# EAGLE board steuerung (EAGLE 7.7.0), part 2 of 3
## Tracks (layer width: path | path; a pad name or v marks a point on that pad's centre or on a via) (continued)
N$60 (continued)
  Bottom 0.2: 6.9,17.2 6.8,17.2 | 6.8,17.2 6.8,17.1 | 6.8,17.1 6.8,16 7.4,16 7.4,25.4 | 7.4,25.4 7.4,25.6 | 30.1,24.9 30.1,25.6 | 30.1,25.6 7.4,25.6 | 7.4,25.6 7.1,25.6 | 7.1,25.6 7.1,17.4 6.8,17.1 | 6.8,17.2 6.8,25.6 7,25.6 | 7,25.6 7,16.2 6.9,16.1 7.2,16.1 7.3,16.2 7.3,17.1 | 7.3,17.2 7.3,17.1 | 7.3,17.1 7.2,17 | 7.2,17 7.2,16.2 | 7.2,17 7.2,24.6 | 7.2,24.6 7.2,25.2 | 7.2,25.2 7.2,25.4 7.3,25.5 7.1,25.5 7,25.6 | 7,25.6 7.1,25.6 | 30.1,25.6 30,25.5 29.7,25.5 29.7,25.3 | 30.1,25.6 30.3,25.6 30.3,22 | 30.3,22 29.9,22 | 29.9,22 29.7,22 | 29.7,22 29.7,22.3 | 29.7,22.3 29.7,22.7 | 29.7,22.7 29.7,25.1 | 29.7,25.1 29.7,25.3 | 29.7,25.3 29.8,25.2 | 29.8,25.2 29.8,24.7 | 29.8,24.7 29.8,22.4 | 29.8,22.4 29.8,22.1 | 29.8,22.1 29.9,22.1 30,22.2 30,23.2 30.1,23.3 | 30.1,23.3 30.1,22.1 | 30.1,23.3 30.1,24.9 | 30.1,24.9 29.8,25.2 | 29.8,25.4 29.8,25.2 | 29.8,25.2 29.7,25.1 | 29.7,25.1 7.3,25.1 7.2,25.2 | 7.2,25.2 7.4,25.4 | 7.4,25.4 29.9,25.4 | 29.8,22.4 29.7,22.3 | 29.7,22 29.7,21.7 | 29.7,21.7 30.3,21.7 | 30.3,21.7 30.3,22 | 30.3,22 30.2,22.1 30.2,22 30.1,21.9 | 29.8,22.1 29.8,21.9 29.9,21.8 30.1,21.8 | 29.9,22 29.9,21.9 29.7,21.7 | 29.7,21.7 29.7,21.6 | 29.7,21.6 30.3,21.6 30.3,21.7 | 29.3,25.2 29.8,24.7 | 7.2,24.6 7.8,25.2 | 29.9,23 29.9,22.9 29.7,22.7 | 29.7,21.6 29.7,21 29.6,20.9 | 29.6,20.9 25.4,20.9 | 25.3,20.9 25.2,20.9 | 24.8,21.3 24.6,21.5 24.6,22 22.9,22 | 22.9,22 22.9,20.4 24.3,20.4 | IC2.11 7.2,25.2 9.1,25.3 29.96,25.3 IC6.3 30.3,22.55 30.3,21.3 | R5.2 23.62,21.08 23.9,20.8 | 24,20.7 24.3,20.4 | 24.3,20.4 30,20.4 30.1,20.4 30.3,20.6 30.3,21.3 | 30.3,21.3 30.1,21.5 29.9,21.5 29.8,21.4 29.8,20.6 29.9,20.5 | 29.9,20.5 30,20.5 30.1,20.6 30.1,21.3 30,21.4 30,20.7 29.9,20.6
  Bottom 0.2: 29.9,20.6 29.9,20.7 | 29.9,20.7 29.9,20.9 29.6,20.9 | 25.2,20.9 25,20.9 | 25,20.9 23.9,20.9 23.9,20.8 | 23.9,20.8 24,20.7 | 24,20.7 24.2,20.7 | 24.8,20.7 29.9,20.7 | 29.9,20.6 29.9,20.5 | 29.9,20.5 24.4,20.5 24.2,20.7 | 24.2,20.7 24.8,20.7 | 24.8,20.7 25,20.9 | 25,20.9 25,21 24.5,21.5 24.5,20.9 24.6,20.8 24.9,20.8 | 25,20.8 24.9,20.8 | 24.9,20.8 24.4,21.3 24.6,21.3 24.9,21 24.8,21 24.4,21.4 24.4,21.7 24.5,21.8 23.1,21.8 | 23.1,21.8 22.9,22 | 22.9,22 22.9,22.1 | 22.9,22.1 24.7,22.1 | 24.7,22.1 24.8,22 24.8,21.3 | 24.8,21.3 25.2,20.9 | 24.7,22.1 25,22.1 25.1,22 | 25.1,22 25.1,21.2 25.4,20.9 | 25.4,20.9 25.3,20.9 | 25.3,20.9 25,21.2 25,21.9 24.9,22 | 23.1,21.8 23.1,21.9 22.9,22.1 | 22.9,22.1 22.9,22.3 25.1,22.3 25.2,22.2 25.2,21 25.4,20.8 | 25.1,22 25.1,22.2
N$61
  Bottom 0.2: 4.6,18.8 4.3,18.8 4.2,18.9 | 4.2,18.9 4.2,19 | 4.2,19 4.8,19 | 4.8,19 4.8,16 3.5,16 3.5,19 | 3.5,19 3.8,19 | 3.8,19 4.4,19 4.5,18.9 4.5,18.6 | 4.5,18.6 4.5,16.3 4.6,16.2 | 4.6,17 4.6,16.2 | 4.6,16.2 4.7,16.1 3.7,16.1 3.6,16.2 3.6,18.8 3.7,18.9 3.9,18.9 | 4,18.9 4.1,18.9 4.2,18.8 4.2,16.2 4.4,16.2 4.4,18.6 4.3,18.7 4,18.7 | 3.9,18.7 3.8,18.7 3.8,16.3 3.7,16.2 3.9,16.2 4,16.3 4,18.7 | 4,18.7 3.9,18.7 | 3.9,18.7 3.8,18.8 3.7,18.8 3.7,16.6 4.1,16.2 | 4.4,18.7 4.5,18.7 4.8,19 | 4.8,19 4.8,21 3.5,21 3.5,20.7 | 3.5,19 3.5,20.7 | 3.5,20.7 3.7,20.9 4.5,20.9 4.6,20.8 4.6,18.7 4.5,18.6 | 4.5,18.6 4.1,18.6 3.6,19.1 3.6,20.6 3.7,20.7 4.1,20.7 | 4.2,20.7 4.4,20.7 | 4.4,20.7 4.5,20.7 4.7,20.9 4.6,20.9 4.4,20.7 | 4.4,20.7 4.4,19.1 4.2,18.9 | 4.2,19 4.2,20.7 | 4.2,20.7 4.1,20.7 | 4.1,20.7 4,20.8 4,18.9 | 4,18.9 3.9,18.9 | 3.9,18.9 3.8,19 | 3.8,19 3.8,20.6
N$62
  Bottom 0.2: 29.9,24.8 29.8,24.8 29.4,25.2
N$63
  Bottom 0.2: 8.3,17.8 8.3,17.3 8.1,17.1 | 8.1,17.1 8.1,16.2 | 8.1,16.2 8.1,16 8.7,16 8.7,24.5 | 29,23 29,22 | 29,22 28.4,22 | 28.4,23.5 28.4,24 | 28.4,24 28.4,24.5 | 28.4,24.5 28.7,24.5 | 28.7,24.5 29,24.5 29,22.8 28.9,22.7 28.9,24.3 28.8,24.4 28.7,24.4 28.5,24.2 28.5,23.8 28.6,23.7 | 28.6,23.7 28.6,24 | 28.6,24 28.6,24.1 | 28.6,24.1 28.8,24.3 28.8,24.1 | 28.8,24.1 28.8,23.9 | 28.8,23.9 28.8,23.8 | 28.8,23.8 28.7,23.7 28.7,24.5 | 28.4,24.5 8.7,24.5 | 8.7,24.5 8.2,24.5 8.2,16.2 8.3,16.1 8.2,16.1 8.1,16.2 | 8.1,17.1 8.1,24.5 8.4,24.5 8.5,24.4 8.5,24.3 | 8.5,24.3 8.5,16.2 8.6,16.1 8.5,16.1 8.4,16.2 8.4,23.3 8.4,23.4 | 8.4,23.4 8.4,24.4 | IC2.12 8.46,24.07 9.9,24.3 | 9.9,24.3 28.69,24.3 IC6.2 | 8.5,24.3 9.9,24.3 | 28.6,24.1 28,24.1 | 28,24.1 8.6,24.1 8.6,24 28.4,24 | 28.4,24 28.6,24 | 28.6,23.7 28.6,23.2 28.5,23.1 | 28.5,22.9 28.4,22.8 | 28.4,22 28.4,21.7 29,21.7 | 29,21.7 29,22 | 29,22 28.9,22.1 28.7,22.1 28.5,21.9 | 28.5,21.9 28.8,21.9 28.9,21.8 | 28.8,24.1 28.5,24.1 28.4,24 | 28.4,22.8 28.4,22 | 28.4,22.8 28.4,23.5 | 28.4,23.5 28.6,23.7 | 28.6,23.7 28.8,23.9 | 28.8,23.8 28.8,23.2 28.7,23.1 | 29,21.7 29,21.6 28.4,21.6 28.4,21.8 28.5,21.9 | 28.6,23.7 28.4,23.7 28,24.1 | 8.4,23.4 9.2,24.2
N$64
  Bottom 0.2: 27.4,23.3 27.2,23.3 27.1,23.4 | 27.1,23.4 27.7,23.4 27.7,23.3 | 27.7,23.3 27.7,21.7 | 27.7,21.7 26.2,21.7 | 26.2,21.7 26.2,23.3 | 26.2,23.3 26.2,23.4 | 26.2,23.4 26.4,23.4 | 26.4,23.4 26.5,23.4 | 27.7,23.3 27.6,23.2 26.4,23.2 26.3,23.3 26.3,23.1 | 26.3,22 26.3,21.8 27.4,21.8 27.5,21.9 | 27.5,21.9 27.5,22.3 | 27.5,22.3 27.5,22.7 27.4,22.7 27.2,22.9 | 27.2,22.9 27,23.1 26.3,23.1 | 26.3,23.1 26.3,23 | 26.3,23 26.3,22 | 26.3,22 26.4,21.9 27.5,21.9 | 27.5,21.9 27.6,21.8 27.6,22.2 27.5,22.3 | 27.5,22.3 26.4,22.3 26.4,22.2 26.5,22.1 | 26.5,22.1 27.4,22.1 | 26.5,22.1 26.4,22.1 26.4,22.5 | 26.4,22.5 26.4,22.7 26.9,22.7 27,22.8 27,22.5 26.5,22.5 | 26.8,23 26.4,23.4 | 26.2,23.4 9.7,23.4 | 9.7,23.4 9.6,23.4 | 9.6,23.4 9.5,23.3 9.5,16 | 9.5,16 9.4,16 9.4,23.4 9.6,23.4 | 9.7,23.4 9.7,16.2 9.5,16 | 9.5,16 9.9,16 9.9,21.7 | 9.9,23.3 9.9,23.2 | 9.9,23.2 9.9,21.7 | 9.9,21.7 9.6,21.4 9.6,16.3 9.8,16.1 | 27.2,22.9 26.4,22.9 | 26.4,22.9 26.3,23 | 26.3,23 10.3,23 | 10.3,23 9.8,23 9.8,23.1 9.9,23.2 | 9.9,23.2 26.1,23.2 26.3,23 | 26.4,22.9 9.8,22.9 | 26.2,23.3 26.4,23.3 26.5,23.4 | 26.5,23.4 27.1,23.4 | 26.2,21.7 26.2,21.6 27.7,21.6 27.7,21.7 | 25.8,23.1 26.4,22.5 | 9.8,22.4 9.8,22.5 10.3,23
N$65
  Bottom 0.2: 28.7,22.6 28.7,22.3 | 28.7,22.3 28.5,22.1 28.5,22.2 28.6,22.3 28.7,22.3 | 28.7,22.3 28.8,22.2 28.8,22.5
N$66
  Bottom 0.2: 30.2,21.9 30.2,21.8
N$67  (via drill 0.6)
  Bottom 0.2: 12.1,18.6 12.1,18.8 | 12.1,18.8 12.2,18.9 | 12.2,18.9 12.3,19 | 12.4,18.7 12.4,16.9 | 12.4,16.2 12.4,16 11.9,16 11.9,19.1 | 11.9,19.1 12,19.1 | 12,19.1 12.4,19.1 | 12.4,19.1 12.4,19 | 12.4,19 12,18.6 12,16.1 12.3,16.1 12.4,16.2 | 12.4,16.2 12.4,16.9 | 12.4,16.9 12.2,17.1 12.2,16.4 12.1,16.3 12.3,16.3 | 12.1,18.8 12.1,19 12.3,19 | 12.3,19 12.4,19.1 | 12.4,19 12.4,18.7 | 12.4,18.7 12.3,18.6 | 11.9,19.1 11.9,20.4 12.2,20.7 12.9,20.7 | 12.9,20.7 12.9,20 | 12.9,20 12.9,19.9 12.6,19.9 12.4,19.7 | 12.4,19.7 12.4,18.8 12.3,18.7 12.3,19.8 12.5,20 12.6,20 | 12.6,20 12.7,20.1 12.7,20.2 | v12.7,20.3 12.7,20.5 12.8,20.6 12.3,20.6 12.1,20.4 12.1,20 | 12.1,19.3 12.1,20 | 12.1,20 12.2,20.1 | 12.4,20.3 12.6,20.5 12.4,20.5 12.4,20.3 | 12.4,20.3 12.2,20.1 | 12.2,20.1 12.2,19.8 v12.7,20.3 | v12.7,20.3 12.7,20.2 | 12.7,20.2 12.9,20 | 12.9,20 12.6,20 | 12.6,20 12.2,20.4 12.5,20.4 12.6,20.3 12.3,20.3 12.2,20.2 12.3,20.1 | 12.2,19.7 12.2,19.5 | 12.2,19.5 12.2,19.1 | 12.2,18.9 12.2,19.1 | 12.2,19.1 12.1,19.2 | 12,19.4 12,19.1 | 12.2,19.5 12.4,19.7 | 12.4,19.7 13,19.7 13.2,19.9 13.2,20.7 12.9,20.7
N$68
  Bottom 0.2: 11,18.8 11,19.1 | 11,19.1 10.9,19.1 | 10.9,19.1 10.8,19.1 | 10.8,19.1 10.6,19.1 | 10.6,19.1 10.6,16 11.2,16 11.2,19.1 | 11.2,19.1 11,19.1 | 10.9,19.1 10.9,16.4 10.7,16.2 | 10.7,16.2 10.7,17.1 10.9,17.1 11,17 11,16.2 | 10.7,16.2 11,16.2 | 11,16.2 11.1,16.1 | 10.6,19.1 10.6,20.7 | 10.6,20.7 11.2,20.7 11.2,20.4 | 11.2,19.1 11.2,20.4 | 11.2,20.4 11.1,20.5 10.8,20.5 10.8,19.3 11.1,19.3 11.1,20.2 10.7,20.6 | 10.7,20.6 10.7,19.2 10.8,19.1 | 10.8,19.1 10.8,19.9 10.9,20 | 10.9,20 10.9,19.4 | 10.9,20 10.9,20.2 | 10.7,20.6 10.6,20.7 | 10.6,20.7 10.6,22.2 10.7,22.3 12.9,22.3 | 12.9,22.3 12.9,21.3 | 12.9,21.3 12.7,21.3 | 12.7,21.3 11.7,21.3 11.2,20.8 10.8,20.8 10.8,22.1 12.7,22.1 12.8,22.2 12.8,22 | 12.8,22 12.8,21.6 | 12.8,21.6 12.7,21.5 12,21.5 | 12,21.5 11.6,21.5 11.1,21 10.9,21 10.9,21.8 11,21.9 | 11,21.9 12.6,21.9 | 12.6,21.9 12.6,21.7 12.5,21.7 | 12.5,21.7 11.1,21.7 11.1,21.5 | 11.1,21.2 11.2,21.2 11.6,21.6 11.2,21.6 | 11.2,21.6 11.1,21.5 | 11.1,21.5 11.1,21.2 | 11.1,21.2 11,21.1 11,21.9 | 12.6,21.9 12.7,21.9 12.8,22 | 12.8,21.6 12.8,21.4 11.2,21.4 | 11.2,21.4 11.2,21.6 | 11.2,21.6 10.7,22.1 10.7,20.8 11.1,20.4 11.1,20.6 | 12.5,21.7 12.6,21.6 | 11.7,21.6 11.7,21.4 11.2,20.9 11.2,21.4 | 11.1,20.6 11.1,20.7 12,21.6 | 12,21.5 11.1,20.6 | 12.9,22.3 13.2,22.3 13.2,21.3 12.9,21.3 | 12.7,21.3 12.7,21.8 13.1,22.2 13.1,21.5 13,21.4
N$69
  Bottom 0.2: 23.3,14.3 23.2,14.3 23,14.5 22.5,14.5 | 22.5,14.5 22.5,14 25.1,14 | 25.1,14 25.1,14.7 | 25.1,14.7 22.5,14.7 22.5,14.5 | 22.5,14.5 22.7,14.7 24.9,14.7 25,14.6 24.5,14.6 24.1,14.2 | 25.1,14.7 27.4,14.7 27.8,14.4 27.8,12.1 27.4,12.1 27.1,12.4 27.1,13.7 26.8,14 | 26.8,14 25.2,14 | 25.1,14 25.2,14 | 25.2,14 25.4,14.2 26.9,14.2 27.1,14 27.1,12.6 27.4,12.3 27.5,12.3 27.6,12.2 27.6,14.4 27.4,14.6 25.1,14.6 25,14.5 26.8,14.5 27.3,14 | 26.8,14 27.3,14 | 27.3,14 27.3,12.7 | 27.3,12.7 27.5,12.5 27.5,12.8 27.4,12.8 27.3,12.7 | 27.3,12.7 27.3,12.5 27.4,12.4
N$70
  Bottom 0.2: 17.9,12.9 17.6,12.9 17.5,12.8 | 19.5,12.8 20,12.8 | 20,12.8 20,13.3 17.5,13.3 17.5,12.8 | 17.5,12.8 19.5,12.8 | 19.5,12.8 19.9,13.2 19.9,13.1 19.8,13 | 19.5,13 19.8,13 | 19.8,13 20,12.8 | 20,12.8 20.1,12.8 21.3,14 | 21.3,14 21.3,14.4 | 28.1,15.5 28.7,15.2 | 28.7,15.2 28.5,15.2 | 28.5,15.2 28.5,14.9 | 28.5,14.5 28.5,12.4 28.4,12.4 28.4,15.2 28.1,15.5 | IC6.17 28.7,15.2 | 28.7,15.2 28.7,15.5 | 28.1,15.5 27.9,15.5 | 21.3,15.5 21.2,15.5 | 21.2,15.5 21.2,14 20.5,13.3 18.96,13.3 IC4.7 | 28.1,15.5 28.3,15.5 | 28.8,15.5 29,15.5 29,12.1 28.4,12.1 28.4,12.3 28.9,12.3 | 28.9,12.3 28.9,12.2 | 28.9,12.3 28.9,15.4 28.8,15.5 | 28.8,15.5 28.7,15.5 | 28.7,15.5 28.5,15.5 | 28.5,15.5 28.5,15.3 | 28.5,15.3 28.6,15.2 | 28.5,15.3 28.3,15.5 | 28.3,15.5 28.5,15.5 | 28.5,15.5 28.6,15.4 28.6,14.7 | 28.6,14.4 28.6,12.6 28.7,12.5 | 28.7,12.5 28.7,12.6 28.8,12.7 28.8,12.5 28.7,12.4 28.7,12.5 | 21.4,15.5 21.3,15.4 | 21.3,15.4 21.3,15.3 | 21.3,15.2 21.3,15.1 | 21.3,14.4 20.1,13.2 20.1,13 21.1,14 21.1,15.5 21.2,15.5 | 21.3,15.2 21.3,15.3 | 21.3,15.3 21.6,15.5 | 21.3,15.2 21.5,15.2 | 21.5,15.2 21.7,15.5 | 21.7,15.5 22,15.5 | 22,15.5 27.8,15.5 | 27.8,15.5 27.9,15.5 | 27.9,15.5 28.5,14.9 | 28.5,14.9 28.5,14.8 | 28.5,14.8 28.5,14.5 | 28.5,14.5 28.6,14.4 | 28.6,14.4 28.6,14.7 | 28.6,14.7 28.5,14.8 | 27.9,15.4 27.8,15.5 | 21.3,14.4 21.3,15.1 | 21.3,15.1 21.6,15.4 | 21.6,15.4 21.7,15.5 | 21.7,15.5 21.6,15.5 | 21.6,15.5 21.4,15.5 | 21.4,15.5 21.3,15.5 | 21.3,15.5 21.3,15.4 | 21.3,14 21.5,14.2 21.5,15.1 22,15.5 | 21.5,15.2 28.5,15.2 | 21.6,15.4 22,15.4 | 22,15.4 27.9,15.4 | 27.9,15.4 28.5,14.8 | 22,15.4 21.4,14.8
N$83  (via drill 0.6)
  other vias: 11.3,21.8
N$84
  Bottom 0.2: 23.6,14.3 22.6,14.3 22.6,14.1 23.3,14.1 23.4,14.2
N$85
  Bottom 0.2: 70.3,9.1 70.3,11.1 | 70.3,11.7 70.3,12 | 70.3,12 70.3,12.1 69.2,12.1 69.2,12 70.4,10.8 70.4,11.9 70.3,12 | 70.3,12 69.4,12 70.3,11.1 | 70.3,11.1 70.3,11.2 | 70.3,11.6 70.3,11.7 | 70.3,11.7 70.2,11.8 69.7,11.8 70.3,11.2 | 70.3,11.2 70.3,11.5 | 70.3,11.5 70.3,11.6 | 70.3,11.6 70.2,11.7 70.1,11.7 70,11.6 70.2,11.6 70.3,11.5
N$86
  Bottom 0.2: 69.2,14 69.2,12.2
N$87
  Bottom 0.2: 22.6,10.4 22.6,10 22.7,9.9 23.2,9.9 | 23.3,9.9 23.2,9.9 | 23.2,9.9 22.8,10.3 22.8,10.2
N$88
  Bottom 0.2: 28.2,3.7 28.3,3.7 28.9,3.1
N$89
  Bottom 0.2: 34.2,26.6 33.9,26.6 | 33.7,26.6 33.6,26.6 33.6,26 | 33.9,25.5 33.8,25.5 33.7,25.6 33.7,23.3 33.6,23.2 33.8,23.2 33.9,23.3 | IC1.5 46.3,20.84 | 46.3,20.84 46.94,20.84 47,20.9 | 47,20.9 47.1,21 | 47.2,21.1 44.2,21.1 | 44.2,21.1 44.2,21 | 44.2,21 44.2,20.8 | 44.2,20.8 44.2,20.6 47.1,20.6 47.2,20.7 44.6,20.7 44.3,21 44.8,21 | 46.9,21 47.1,21 | 47.1,21 47.2,21.1 | 47.2,21.1 47.2,20.6 44.4,20.6 44.2,20.8 | 44.2,20.8 44.6,20.8 44.8,21 | 44.8,21 46.9,21 | 46.9,21 47,20.9 | 47,20.9 47.1,20.8 44.5,20.8 44.2,21.1 | IC6.6 33.77,23.23 33.5,23.5 | 33.5,23.5 33.5,21.6 34.1,21.6 34.1,23.5 | 34.1,23.5 33.5,23.5 | 33.5,23.5 33.5,25.6 | 33.5,25.6 33.7,25.8 33.9,25.8 | 39.2,25.8 38.5,26.5 34.1,26.5 34.1,23.5 | 39.2,25.8 40.3,24.7 40.3,21 40.4,20.9 42.9,20.9 43.2,20.6 46.06,20.6 46.3,20.84 | 44.2,21.1 44.1,21.1 | 40.8,21.1 40.6,21.3 40.6,24.8 38.7,26.7 33.5,26.7 33.5,26.1 | 33.5,26.1 33.5,25.8 | 33.5,25.6 33.5,25.8 | 33.5,25.8 33.6,25.9 | 33.6,25.9 33.7,26 | 39.2,26 39.3,25.9 39.3,25.8 | 39.3,25.8 40.4,24.7 40.4,24.8 39.4,25.8 39.4,25.7 40.5,24.6 40.5,21.2 40.4,21.1 40.8,21.1 | 40.8,21.1 44.1,21.1 | 44.1,21.1 44.2,21 | 44.2,21 43,21 | 42.9,21 43,21 | 43,21 43.2,20.8 44.2,20.8 | 33.8,23.3 33.9,23.3 | 33.9,23.3 34.1,23.5 | 33.9,23.3 33.9,25.7 | 33.9,25.7 34,25.8 33.9,25.8 | 33.9,25.8 33.8,25.7 | 33.6,25.9 33.6,26 | 33.6,26 33.5,26.1 | 39.2,25.8 39.3,25.8 | 39.3,25.8 39.4,25.9 39.2,25.9 38.5,26.6 38.7,26.6 39.2,26.1 | 33.6,26 33.9,25.7 | 33.9,26 33.9,26.6 | 33.9,26.6 33.7,26.6 | 33.7,26.6 33.7,26 | 33.7,26 33.8,25.9 | 33.9,25.7 33.9,26 | 33.9,26 34.5,26.6
N$90
  Bottom 0.2: 10.8,19 10.8,18.8
N$92
  Bottom 0.2: 51.4,14.3 51.7,14.3 52,14 52,10.9 52.1,10.8 52.2,10.8 52.5,11.1 | 52.5,11.1 52.5,13.9 52.4,14 52.4,11.2 52.3,11.1 52.5,11.1 | 52.5,11.1 52.8,11.4 52.8,13.6 52.7,13.7 52.7,11.5 52.6,11.4 52.9,11.4 53.1,11.6 53.1,13.3 52.9,13.5 52.9,11.7 53,11.6 53.4,12 53.4,12.9 53.3,13 53.3,12.1 53.2,12 53.2,13.1
N$93
  Bottom 0.15: 32.5,22.4 32.4,22.4 32.4,21.8 32.5,21.8 32.5,22.4 | 32.5,22.4 32.6,22.4 | 32.7,22 32.6,22 32.6,22.4 | 32.6,22.4 32.7,22.4 32.7,22.1
N$94
  Bottom 0.2: 59.8,21.6 61.2,23
N$95
  Bottom 0.2: 66,15.4 65.6,15 65.8,15 65.9,15.1 65.5,15.1 65.4,15
N$96
  Bottom 0.2: 32.7,2 35.4,2 35.4,1.8 | 35.4,1.8 35.3,1.7 32.8,1.7 32.7,1.8 32.7,1.9 35.3,1.9 35.4,1.8 | 35.4,1.8 35.4,1.6 | 35.4,1.6 35.4,1.5 32.7,1.5 32.6,1.6 32.6,1.2 35.4,1.2 35.4,1.3 35.3,1.4 32.9,1.4 32.8,1.3 32.8,1.6 32.6,1.8 33.5,1.8 34.2,2.5 | 60.5,12.4 65.5,12.4 65.5,12.6 60.4,12.6 | 67.2,13.8 67.1,13.8 66.1,12.8 | 66,12.7 65.4,12.1 65.4,13.8 | 65.4,13.9 65.4,14.6 65.6,14.6 65.6,12.4 65.8,12.6 65.8,13.3 | 55.7,11.4 60.4,11.4 60.4,11.6 | 60.4,11.6 60.4,12.2 | 60.4,12.2 60.4,13.6 | 60.4,13.6 60.4,14.1 | 60.4,14.1 60.4,14.9 | 60.4,14.9 60.3,14.9 | 60.3,14.9 59.1,14.9 59.1,11.5 | 22.9,8.3 22.9,8.5 23.1,8.7 24.4,8.7 24.7,8.4 24.7,8 24.9,7.8 26.1,7.8 26.5,7.4 | 23.5,7.4 26.5,7.4 | 26.5,7.4 26.7,7.2 | 26.7,7.2 27.3,6.6 31,6.6 31.8,5.8 33.6,5.8 | 34.8,3.81 X1.3 34.7,3.9 34.7,5.3 34.5,5.5 33.9,5.5 | C2.1 65.9,14.7 | 65.9,14.7 63.1,14.7 | 60.55,14.7 IC5.3 | IC5.3 59.8,14.4 60.1,14.7 60.55,14.7 | 60.55,14.7 63.1,14.7 | 63.1,14.7 R2.1 | IC5.3 59.8,12.4 | 59.8,12.4 59.8,11.5 | 59.8,11.5 59.4,11.5 | 59.4,11.5 59.1,11.5 | 59.1,11.5 58.8,11.5 | 58.8,11.5 55.8,11.5 | 55.8,11.5 55.7,11.5 | 55.7,11.5 52.6,8.4 52.7,8.3 52.7,1.3 | R3.2 23.02,7.78 23.7,7.1 26.3,7.1 27.1,6.3 30.8,6.3 31.6,5.5 | 31.6,5.5 31.7,5.5 | 31.7,5.5 33.7,5.5 | 33.6,5.8 33.9,5.5 | 33.9,5.5 33.7,5.5 | 33.7,5.5 33.6,5.6 31.8,5.6 31,6.4 30.9,6.4 | 30.9,6.4 27.4,6.4 | 27.4,6.4 27.2,6.4 26.4,7.2 | 26.4,7.2 26.6,7.2 27.4,6.4 | 26.4,7.2 24.2,7.2 23.7,7.7 23.7,7.5 24,7.2 | 26.7,7.2 26.5,7.2 26.1,7.6 24,7.6 23.9,7.7 23.9,8.6 24.3,8.6 24.4,8.5 24.4,7.8 24.5,7.7 24.9,7.7 24.6,8 24.6,8.4 24.5,8.5 24.5,7.5 24,7.5 23.7,7.2 23.7,8.2 24,8.5 24.2,8.5 24.3,8.4 24.3,8.2 | 24.3,7.7 24.3,8.2
  Bottom 0.2: 24.3,8.2 24.1,8.4 24.1,7.9 24,7.8 24.2,7.8 | 30.9,6.4 30.9,6.3 31.7,5.5 | 31.6,5.5 32.5,4.6 | 32.5,4.6 32.5,2.3 | 32.5,2.3 32.5,2.1 | 32.5,2.1 35.5,2.1 | 35.5,2.1 35.5,3.8 | 35.5,4.2 35.5,4.5 | 35.5,4.5 35.5,4.9 | 35.5,4.9 35.5,5.5 35.4,5.6 32.1,5.6 31.9,5.4 32.6,4.7 32.6,5.4 32.1,5.4 32.4,5.1 | 32.4,5.1 32.4,5.3 | 32.4,5.1 32.4,5 32.5,4.9 32.5,4.6 | 32.5,2.3 32.6,2.2 33.8,2.2 33.8,5.3 33.7,5.4 32.8,5.4 32.7,5.3 32.7,2.3 33.6,2.3 33.7,2.4 32.9,2.4 32.9,5.1 32.8,5.2 33.6,5.2 33.6,2.6 33.7,2.5 33.7,5.2 33.6,5.3 33.2,5.3 33,5.1 33,2.5 33.5,2.5 33.5,5.1 33.3,5.1 | 33.3,5.1 33.2,5.1 33.1,5 33.1,2.7 33.2,2.7 33.3,2.6 33.3,5.1 | 35.5,2.1 35.5,1.3 | 35.5,1.3 35.5,1.1 35.7,1.1 | 35.9,1.1 51.5,1.1 | 51.8,1.1 51.9,1.1 | 51.9,1.1 52.3,1.1 | 52.5,1.1 52.6,1.1 52.7,1.2 | 52.7,1.2 52.7,1.3 | 32.5,2.1 32.5,1 37.8,1 | 38,1 52.8,1 52.9,1.1 52.9,8.5 55.8,11.4 55.8,11.5 | 55.7,11.5 55.6,11.5 52.6,8.5 52.6,1.4 52.3,1.1 | 52.3,1.1 52.5,1.1 | 52.5,1.1 52.7,1.3 | 52.7,1.2 52.7,1.1 | 59.8,11.5 60.2,11.5 60.3,11.6 60.3,12.6 | 60.3,12.6 60.3,14.9 | 60.4,14.9 60.6,14.9 | 60.6,14.9 60.6,14.5 | 60.6,14.5 60.6,13.8 | 60.6,13 60.6,12.8 | 60.6,12.8 60.6,11.4 | 60.6,11.4 59.5,11.4 59.4,11.5 | 59.4,11.5 59.3,11.6 59.3,13.2 59.4,13.3 60.1,13.3 60.2,13.2 | 60.2,12 60.2,11.7 59.5,11.7 59.5,13 59.7,13 | 59.7,13 60,13 60.2,13.2 | 60.2,13.2 60.2,13.1 | 60.2,13.1 60.2,12 | 60.2,12 60,11.8 60,13.2 59.9,13.2 59.7,13 | 59.7,13 59.7,11.9 59.4,11.6 | 59.8,12.4 59.7,12.4 58.8,11.5 | 60.6,14.9 65.2,14.9 | 65.2,14.9 66.3,14.9 | 60.1,11.6 60.4,11.6 | 60.4,11.6 60.6,11.4 | 60.6,11.4 61.7,11.4 62.3,12 65.6,12 67.4,13.8 | 67.4,13.8 67.4,15.5 65.8,15.5 65.2,14.9 | 65.8,13.3 65.8,14.5
  Bottom 0.2: 65.8,14.5 65.8,14.6 65.9,14.7 | 65.9,14.7 65.9,13.5 | 65.9,12.8 65.9,12.9 | 65.9,13.1 65.9,13.5 | 65.9,13.5 66.1,13.7 | 66.1,13.7 66.5,13.7 | 66.5,13.7 66.7,13.7 | 66.7,13.7 66.8,13.8 | 66.7,13.7 65.9,12.9 | 65.9,12.9 65.9,13.1 | 65.9,13.1 66.3,13.5 66.1,13.5 | 66.1,13.5 66.1,12.8 | 66.1,12.8 66,12.7 | 66,12.7 66.1,12.7 | 66.1,12.7 67.2,13.8 | 67.2,13.8 67.1,13.9 67,13.9 66,12.9 66,13.2 66.5,13.7 | 66.5,13.7 66.2,14 66.2,13.8 66.1,13.7 | 60.4,11.6 61.8,11.6 | 61.8,11.6 61.9,11.7 | 61.9,11.7 62,11.8 | 62,11.8 62.2,12 60.6,12 60.5,12.1 60.5,11.8 62,11.8 | 60.4,12.2 65.6,12.2 | 60.3,12.6 60.4,12.6 | 60.4,12.6 60.6,12.8 | 60.6,12.8 65.7,12.8 65.5,13 60.6,13 | 60.6,13 60.3,13 60.2,13.1 | 60.2,13.1 60.3,13.1 60.5,13.3 65.8,13.3 | 65.8,13.3 65.7,13.2 60.8,13.2 60.6,13 | 60.6,13 60.6,13.4 | 60.6,13.4 60.4,13.6 | 60.4,13.6 66,13.6 66.1,13.5 | 66.1,13.5 60.7,13.5 60.6,13.4 | 60.6,13.4 60.6,13.8 | 60.6,13.8 65.4,13.8 | 65.4,13.8 65.4,13.9 | 65.4,13.9 65.5,14 60.5,14 60.4,14.1 | 60.4,14.1 60.5,14.2 65.4,14.2 65.5,14.1 65.5,14.3 60.5,14.3 60.5,14.4 60.6,14.5 | 60.6,14.5 65.8,14.5 | 35.4,1.6 35.6,1.4 | 35.9,1.1 35.7,1.1 | 35.7,1.1 35.5,1.3 | 33.6,5.8 35.4,5.8 35.6,5.6 | 35.6,5.6 35.6,5.3 | 35.6,5.3 35.6,4.6 | 35.6,4.6 35.6,1.4 | 35.6,1.4 35.8,1.2 | 35.8,1.2 35.9,1.1 | 66.1,12.8 66.1,12.7 | 66.1,12.7 65.6,12.2 | 65.6,12.2 65.6,13.3 66.1,13.8 | 61.6,11.5 61.7,11.5 61.8,11.6 | 62,11.8 67.3,11.8 67.3,12.1 | 67.3,12.1 67.3,13.9 67.4,13.8 | 67.4,13.8 67.4,11.8 65.7,11.8 65.6,11.9 67.2,13.5 67.2,13.2 | 67.2,13.2 67.2,12.1 | 67.2,12.1 67.1,12 66.9,12 | 66,12 65.9,12 65.8,11.9 67.1,11.9 67.2,12 67.2,12.1 | 67.1,13.1 66,12 | 66,12 66.9,12 | 66.9,12 67.1,12.2 67.1,13.1 | 67.1,13.1 67.2,13.2
  Bottom 0.2: 67.2,13.2 67,13.2 65.9,12.1 66.8,12.1 67,12.3 67,12.4 | 67,12.4 67,12.8 66.9,12.8 66.3,12.2 66.7,12.2 66.8,12.3 66.8,12.5 66.9,12.6 66.8,12.6 66.5,12.3 66.9,12.3 67,12.4 | 51.9,1.1 51.9,7.9 55.5,11.5 55.5,11.3 52.1,7.9 52.1,1.3 52.2,1.2 52.2,7.9 52.4,8.1 52.4,1.9 | 52.4,1.9 52.4,1.3 52.2,1.3 52.1,1.2 52.1,1.6 52.4,1.9 | 52.4,1.9 52.3,1.9 51.5,1.1 | 51.5,1.1 51.8,1.1 | 51.8,1.1 52,1.3 | 35.6,5.6 37.3,3.9 | 37.3,3.9 37.3,3.8 37.4,3.7 37.4,3.8 | 37.4,3.8 37.3,3.9 | 37.4,3.8 37.6,3.6 37.6,1.4 38,1 | 38,1 37.8,1 | 37.8,1 37.5,1.3 37.5,3.4 37.4,3.5 | 37.2,3.7 37.1,3.8 | 36.9,4 36.7,4.2 | 36.5,4.4 36.3,4.6 | 36.3,4.6 35.6,5.3 | 35.6,5.3 35.7,5.3 37.5,3.5 37.2,3.5 | 37,3.5 36.9,3.5 | 36.7,3.5 35.6,3.5 35.4,3.7 35.7,3.7 | 37.2,3.7 36.5,3.7 | 36.5,3.7 35.7,3.7 | 35.7,3.7 35.4,4 36.9,4 | 36.9,4 37.1,3.8 | 37.1,3.8 36.4,3.8 | 36.3,3.8 35.5,3.8 | 35.5,3.8 35.5,4.2 | 35.5,4.2 36.7,4.2 | 36.7,4.2 36.5,4.4 | 36.5,4.4 35.6,4.4 35.5,4.5 | 35.5,4.5 35.6,4.6 | 35.6,4.6 36.2,4.6 | 36.3,4.6 36.2,4.6 | 36.2,4.6 36.1,4.7 35.7,4.7 35.5,4.9 | 35.5,4.9 35.6,4.9 35.7,5 35.7,4.6 35.8,4.5 35.8,1.2 | 35.8,1.2 36,1.2 36,3.6 36.2,3.6 36.2,1.2 36.4,1.2 36.4,3.7 36.3,3.8 | 36.3,3.8 36.4,3.8 | 36.4,3.8 36.5,3.7 | 36.5,3.7 36.5,1.2 36.7,1.2 36.7,3.5 | 36.7,3.5 36.9,3.5 | 36.9,3.5 36.9,1.2 37.1,1.2 37.1,3.4 37,3.5 | 37,3.5 37.2,3.5 | 37.2,3.5 37.2,1.3 37.3,1.2 37.4,1.2 37.4,3.5 | 37.4,3.5 37.2,3.7 | 61.5,12.7 61.5,12.1 61.9,11.7 | 61.9,11.7 67.4,11.7 67.4,12 67.3,12.1
N$97
  Bottom 0.2: 61.8,21.1 61.3,20.6
N$98
  Bottom 0.2: 4,5.8 4,7.7 | 4,7.7 3.9,7.7 3.9,5.3 6.1,7.6 6.1,7.7 | 6.1,7.7 4.6,7.7 | 4.1,7.7 4.1,6 | 4.1,5.5 4.1,6 | 4.1,6 5.5,7.5 6,7.5 5.9,7.6 4.7,7.6 | 4.3,7.6 4.1,7.6 4,7.7 | 4,7.7 4.1,7.7 | 4.1,7.7 4.6,7.7 | 4.6,7.7 4.7,7.6 | 4.7,7.6 4.3,7.6 | 4.3,7.6 4.2,7.5 | 4.2,6.4 4.2,5.7 | 4.2,5.6 4.2,5.7 | 4.2,5.7 5.9,7.4 4.4,7.4 4.4,7 | 4.4,7 4.4,6.8 | 4.4,6.6 4.4,6.4 | 4.4,6.4 4.4,6 4.3,5.9 4.3,5.7 6.1,7.7 | 6.1,7.7 5.6,7.3 | 5.1,7.3 4.9,7.3 | 4.7,7.3 4.4,7.3 4.2,7.5 | 4.2,7.5 4.2,6.4 | 4.2,6.4 4.5,6.1 4.5,6.2 5.6,7.3 | 5.6,7.3 5.5,7.3 | 5.5,7.3 5.3,7.3 | 5.3,7.3 4.4,6.4 | 4.4,6.4 4.6,6.4 5.5,7.3 | 5.3,7.3 5.1,7.3 | 5.1,7.3 4.4,6.6 | 4.4,6.6 4.4,6.8 | 4.4,6.8 4.9,7.3 | 4.9,7.3 4.7,7.3 | 4.7,7.3 4.4,7
N$99
  Bottom 0.2: 8.2,6.3 8.2,6 6.5,4.3 6.7,4.3 8.1,5.7 | 8.5,14 8.5,11.1 8.2,10.8 | 8.5,14 8.3,14 | 8.3,14 8.1,14 8.1,10.7 | 8.1,10.7 8.3,10.7 | 8.3,10.7 8.6,10.7 | 8.6,10.7 8.6,14 8.5,14 | 8.3,14 8.3,11.1 8.4,11 | 8.4,11 8.4,10.9 | 8.4,10.9 8.6,10.7 | 8.6,5.4 7.4,4.2 | 8.1,10.7 8.1,5.9 | 8.1,5.4 8.1,5.3 7,4.2 7.3,4.2 8.5,5.4 8.5,10.9 8.4,11 | 8.4,10.9 8.4,10.8 8.3,10.7 | 8.3,10.7 8.3,5.7 | 8.3,5.4 8.3,5.7 | 8.3,5.7 8.1,5.9 | 8.1,5.9 8.1,5.7 | 8.1,5.7 8.1,5.4 | 8.1,5.4 6.9,4.2 7.1,4.2 8,5.1 | 8.6,5.4 8.6,5.2 7.5,4.1 | 8.6,10.7 8.6,5.4
N$100
  Bottom 0.2: 29.7,4.8 29.7,2.8 30.2,2.3 30.2,4.9 29.5,5.6 | 29.5,5.6 29.6,5.6 | 29.6,5.6 30.6,5.6 31,5.2 31,1.1 | 31,1.1 28.9,1.1 | 28.9,1.1 28.9,4.9 29.6,5.6 | 29.5,5.6 29.1,5.6 | 29.1,5.6 28.8,5.6 | 28.8,5.6 28.5,5.3 28.5,4.3 | 28.5,4.3 28.5,1.1 | 28.5,1.1 28.8,1.1 | 28.9,1.1 28.8,1.1 | 28.8,1.1 28.7,1.2 28.7,1.6 | 28.7,5.1 28.7,5.3 | 28.7,5.3 30.7,5.3 30.7,1.8 | 30.7,1.8 30.7,1.3 30.6,1.2 30.8,1.2 30.9,1.3 30.9,5.1 30.5,5.5 30.5,5.1 30.4,5 30.5,5 30.6,4.9 29.2,4.9 29.1,5 | 29.1,5 28.7,5.4 28.7,5.3 | 28.7,5.1 28.7,4.8 | 28.7,4.8 28.7,4.6 | 28.7,4.6 28.7,1.6 | 28.7,1.6 29,1.3 30.5,1.3 30.5,1.7 | 30.5,1.8 30.5,2.3 30.3,2.5 29.9,2.5 | 29.9,2.5 29.5,2.5 29.1,2.1 29.1,1.7 | 29.1,1.7 29.1,1.6 29,1.5 30.6,1.5 30.6,1.7 30.7,1.8 | 30.7,1.8 29.2,1.8 29.1,1.7 | 29.1,1.7 30.5,1.7 | 30.5,1.7 30.5,1.8 | 30.5,1.8 30.6,1.9 29.1,1.9 29,2 29.4,2 29.9,2.5 | 28.5,1.1 28.5,1 31,1 31,1.1 | 31,1.1 30.9,1.2 | 29.1,5 29.1,5.6 | 22.6,11.9 22.5,11.9 22.5,12 | 22.5,12 25.1,12 25.1,11.5 22.5,11.5 | 22.5,11.5 22.5,11.8 24.1,11.8 24.3,11.6 23.73,11.6 | 22.7,11.6 22.6,11.7 | 23.4,11.9 22.6,11.9 | 22.6,11.9 22.5,12 | 22.5,12 22.3,12 22.1,11.8 | 22.2,11.8 22.3,11.8 22.4,11.9 22.4,11.6 | 22.4,11.6 22.5,11.5 | X1.2 28.34,3.77 26,6.2 | 25.9,6.2 21.6,6.2 | 21.6,6.2 21.6,10.7 | 22.3,11.5 22.4,11.6 | 22.4,11.6 22.5,11.6 | 22.7,11.6 23.73,11.6 | 23.73,11.6 IC4.3 | 22.5,11.5 22.3,11.5 | 21.6,10.8 22,11.2 | 22,11.2 22.3,11.5 | 22.4,11.6 22.2,11.8 | 22.2,11.8 22.1,11.8 | 22.1,11.8 22,11.7 22,11.4 | 22,11.2 22,11.4 | 22,11.4 22.2,11.6 | 21.6,10.8 21.6,10.7 | 21.6,10.7 21.5,10.7 | 21.6,10.8 21.5,10.7 | 21.5,10.7 21.5,6.2 21.6,6.2 | 22.7,11.6 22.5,11.6 | 22.5,11.6 21.7,10.8 21.7,6.5 21.8,6.4 | 21.7,6.3 21.8,6.4
  Bottom 0.2: 21.8,6.4 25.6,6.4 | 25.6,6.4 29.2,2.8 | 25.6,6.4 26,6.4 26.6,5.8 | 26.8,5.6 27.4,5 | 27.4,5 28.9,3.5 28.9,3.4 28.8,3.3 28.8,3.4 26,6.2 | 26,6.2 25.9,6.2 | 25.9,6.2 25.8,6.3 | 28.8,5.6 26.8,5.6 | 26.8,5.6 26.6,5.8 | 26.6,5.8 26.6,5.7 26.9,5.4 27.5,5.4 | 28.8,5.4 27.5,5.4 | 27.5,5.4 27.3,5.2 28.6,5.2 28.7,5.1 | 28.7,5.1 27.5,5.1 27.4,5 | 27.4,5 27.7,5 | 27.7,5 28.5,5 28.7,4.8 | 28.7,4.8 28.5,4.8 | 28.5,4.8 27.8,4.8 27.7,4.9 27.7,5 | 28.5,4.8 28.7,4.6 | 28.7,4.6 27.9,4.6 27.8,4.5 28.3,4.5 28.5,4.3 | 28.5,4.3 28.4,4.2 28.4,4.3 27.7,5
N$101
  Bottom 0.2: 9.2,4 9.2,4.1 9,4.3 9,4.4 9.5,4.9 9.5,4.8 9.1,4.4 9.3,4.4 9.3,4.5 9.8,5 | IC2.4 9.73,11.83 9.73,13.97 9.7,14 | 9.7,14 9.4,14 9.4,10.6 | 9.4,10.6 9.9,10.6 | 9.9,10.6 9.9,10.9 | 9.9,10.9 9.9,14 | 9.9,14 9.8,13.9 | 9.8,13.9 9.6,13.9 9.7,14 | 9.7,14 9.9,14 | 9.8,13.9 9.7,13.8 9.5,13.8 9.5,10.8 9.6,10.7 9.8,10.7 | 9.8,10.7 9.8,10.9 | 9.8,10.9 9.8,13.5 9.6,13.7 9.6,10.8 | 9.6,10.8 9.4,10.6 | 9.4,10.6 9.4,4.3 9.8,4.3 9.8,5 | 9.8,5 9.8,10.7 | 9.8,10.9 9.9,10.9 | 9.9,10.6 9.9,4.1 | 9.9,4.1 9.8,4.2 9.6,4.2 9.6,10.8 | JP7.4 9.73,2.33 9.8,2.4 9.8,3.4 9.9,3.5 | 9.9,3.5 9.9,3.1 | 9.9,3.1 9.9,2.4 9.8,2.3 9.6,2.3 9.6,2.8 9.9,3.1 | 9.9,3.5 9.9,4.1 | 9.8,5 9.9,5 10.6,4.3 10.4,4.3 10,4.7 10,4.5 10.1,4.4
N$102
  Bottom 0.2: 11.1,6.3 13.1,4.3 12.8,4.3 11.1,6 11.2,6 12.8,4.4
N$103
  Bottom 0.2: 19.1,19.6 19.3,19.6 19.6,19.3
N$104
  Bottom 0.2: 18.6,6.5 19,6.1 20.6,6.1 21.3,5.4 23.7,5.4 23.8,5.3 23.7,5.3 | 18.4,10.7 17.5,10.7 17.5,10.3 | 17.5,10.3 17.5,9.8 | 17.5,9.8 17.7,9.8 | 17.7,9.8 17.8,9.8 | 17.8,9.8 20,9.8 20,10.7 17.7,10.7 17.6,10.6 17.6,10.2 | 18.6,10.1 19.8,10.1 19.8,10.6 19.9,10.5 19.9,10 17.6,10 17.6,10.2 | 18.6,10.1 18,10.1 | 18,10.1 17.7,10.1 | 17.6,10.2 17.5,10.3 | 25.4,5.6 25.4,5.3 24,5.3 23.8,5.5 | 18,10.1 18,9.6 17.8,9.8 | 17.9,9.3 17.9,9.4 18.6,10.1 | 17.5,9.8 17.5,9.3 18.6,8.2 18.6,6.5 | 18.6,10.1 18.6,6.6 18.9,6.3 20.5,6.3 21.1,5.7 | 21.2,5.6 21.2,5.5 21.1,5.6 21.1,5.7 | 21.1,5.7 21.2,5.6 | 21.3,5.5 21.2,5.6 | 21.2,5.6 22,5.6 | 23.5,3.2 23.5,2.1 25.5,2.1 25.5,5.5 25.5,5.6 | 23.5,4.3 23.5,5 23.2,5.3 22.7,5.3 | 22.6,5.3 21.6,5.3 | 21.2,5.3 20.3,6.2 | 18.4,9.7 18.4,6.7 18.6,6.5 | 17.7,9.8 17.7,9.4 | 17.7,9.4 17.7,9.3 18.3,8.7 18.3,9.6 | 17.6,9.6 17.9,9.6 | 18.3,9.6 18.5,9.6 | 18.3,9.6 17.9,9.6 | 17.9,9.6 17.7,9.4 | 17.7,9.4 18.1,9 18.1,9.2 | 18.1,9.2 18.1,9.4 18.2,9.5 18.2,9.3 18.1,9.2 | 23.5,5.3 23.7,5.3 | 23.7,5.3 23.7,5 | 23.7,3.1 23.7,3.2 | 23.7,3.3 23.7,4.3 | 23.7,4.4 23.7,5 | 23.7,5 23.6,5.1 | 23.6,5.1 23.4,5.3 | 23.6,5.1 23.6,4.8 | 23.6,4.8 23.6,4.3 | 23.6,4 23.6,3.8 | 23.6,3.6 23.6,2.8 23.7,2.7 | 23.9,2.5 23.7,2.7 | 23.7,2.7 23.7,2.3 23.6,2.3 | 21.2,5.3 23.1,3.4 23.1,1.9 25.9,1.9 25.9,5.2 25.5,5.6 | 25.4,5.6 22,5.6 | 22,5.6 21.6,5.2 | 21.6,5.1 21.6,5 23.4,3.2 23.4,2.3 23.3,2.2 23.3,3 23.2,3.1 24.7,3.1 25.7,2.1 25.7,5.2 | 25.7,5.3 25.7,5.2 | 25.7,5.2 25.4,4.9 | 21.2,5.3 21.6,5.3 | 21.6,5.3 23.7,3.2 | 23.7,3.2 23.7,3.3 | 23.7,3.3 21.9,5.1 22.1,5.1 23.6,3.6 | 21.6,5.2 21.9,5.2 | 21.9,5.2 22.2,5.2 | 22.4,5.2 22.9,5.2 | 23.2,5.2 24.2,5.2 24.5,4.9 | 23.6,3.6 23.6,3.8 | 23.6,3.8 22.2,5.2
  Bottom 0.2: 22.2,5.2 22.4,5.2 | 22.4,5.2 23.6,4 | 23.6,4 23.6,4.3 | 23.6,4.3 22.6,5.3 | 22.6,5.3 22.7,5.3 | 22.7,5.3 23.7,4.3 | 23.7,4.3 23.7,4.4 | 23.7,4.4 22.9,5.2 | 22.9,5.2 23.2,5.2 | 23.2,5.2 23.6,4.8 | 23.6,4.8 23.4,4.8 23.2,5 22.8,5 | 22.8,5 22.1,5 21.9,5.2 | 21.6,5.2 21.4,5.2 | 21.6,5.2 21.6,5.1 | 21.6,5.1 23.5,3.2 | 23.5,3.2 23.5,4.3 | 23.5,4.3 22.8,5 | 25.4,5.6 25.5,5.6
N$106
  Bottom 0.2: 18.5,6.9 18.5,6.8 19.1,6.2
N$108
  Bottom 0.2: 5.7,17.6 5.7,16 | 5.7,16 5.9,16 | 5.9,16 6.1,16 6.1,23.2 | 6.1,23.2 5.9,23.4 2.8,23.4 | 2.8,23.4 2.7,23.3 2.7,22.1 2.9,21.9 5.3,21.9 5.6,21.6 5.6,16 5.7,16 | 5.9,16 5.9,22.6 | 5.9,22.6 5.9,22.9 | 5.9,22.9 5.9,23.2 2.9,23.2 2.9,23.1 2.8,23 5.8,23 5.9,22.9 | 5.9,22.9 2.9,22.9 2.8,22.8 5.7,22.8 5.9,22.6 | 5.9,22.6 5.8,22.6 | 2.8,22.6 5.8,22.6 | 5.8,22.6 6,22.4 2.9,22.4 2.8,22.3 5.9,22.3 6,22.2 3.1,22.2 2.8,22.5 2.8,22.1 2.9,22 5.6,22 5.7,21.9 3.1,21.9 2.9,22.1 5.7,22.1 5.8,22 5.8,21.6 | 5.8,18.6 5.8,21.6 | 5.8,21.6 5.6,21.8 | 6.1,23.2 6.1,23.5 | 6.1,23.6 6.1,23.5 | 6.1,23.5 6,23.4 6,23.5 6.1,23.6 | 6.1,23.6 2.6,23.6 2.6,21.9 2.7,21.8 5.3,21.8 5.7,21.4 | 2.8,23.4 2.7,23.5
N$109
  Bottom 0.2: 20,3.1 20,3.3 | 20,3.3 20.8,3.3 | 20,3.3 19.4,3.3 19.9,3.8
N$110
  Bottom 0.2: 17.7,6.3 17.8,6.3 18.7,5.4
N$111  (via drill 0.6)
  Top 0.2: v4.2,22.8 42.1,22.8 v42.1,9.9
  Bottom 0.05: v4.2,22.8 5.8,22.8 IC2.10
  Bottom 0.2: 36.4,13.7 36.4,14.9 36.1,14.9 36.1,13.7 | 36.1,13.7 36.2,13.6 36.2,13.7 | 36.2,13.7 36.2,14.7 36.3,14.8 36.3,13.5 | 36.2,10.8 36.2,12 | 36.2,12 36.2,12.7 | 36.2,12.7 36.3,12.8 36.3,12.6 | 36.4,10.7 36.7,10 | 36.8,10 37.8,9.6 | 37.8,9.6 43.1,9.6 43.1,9.8 43,9.9 37.4,10.2 36.8,10.1 | 36.8,10.1 42.9,9.7 43,9.8 43,9.5 | 36.6,13.6 36.6,15 36,15 36,13.6 | IC6.11 36.6,12.9 36.6,12.5 | 36.6,10.8 36.6,10 | 36.6,10 37.3,10.1 | 37.3,10.1 v42.1,9.9 | 36.6,10.8 37.1,10.3 43,10.3 43.2,10.1 43.2,9.5 43,9.5 | 36.6,10.8 36.6,12.5 | 36.6,12.5 36.4,12.7 36.4,10.7 | 36.4,10.7 36.7,10.4 | 36.7,10.4 36.8,10 | 36.8,10 36.9,10.1 | 36.9,10.1 36.5,10.5 | 36.5,10.5 36.4,10.7 | 36.4,10.7 36.3,12.6 | 36.3,12.6 36.2,12.7 | 43,9.5 37.7,9.5 | 37.7,9.5 36.8,10 | 36.8,10 36.5,10.5 | 36.5,10.5 36.7,10.4 | 36.7,10.4 36.6,10 | 36.6,10 36.7,10 | 36.7,10 36.8,10 | 36.8,10 43.1,10 43,10.1 37.3,10.1 | 37.3,10.1 37.1,10.1 | 37.1,10.1 36.9,10.1 | 36.9,10.1 36.8,10.1 | 36.8,10.1 36.7,10.1 36.7,10.4 | 36.7,10.4 36.8,10.4 | 36.8,10.4 37.1,10.1 | 36.8,10.4 36.7,10.5 36.7,10.4 | 36.7,10.4 36.9,10.2 | 36,13.6 36,12.9 | 36,12.9 36.2,12.7 | 36.2,13.7 36.1,13.7 | 36.1,13.7 36,13.6 | 36,12.9 36,12.2 36.2,12 | 36.2,10.8 36.5,10.5 | 36.9,10.1 37.7,9.5 | 37.7,9.5 37.8,9.6 | 36.2,10.8 36.2,10.4 37.1,9.5 41.3,9.5 41.5,9.7 | 41.5,9.7 37.1,9.7 36.3,10.5 36.4,10.5 37,9.9 41.3,9.9 41.5,9.7
N$112
  Bottom 0.2: 67.2,10.4 67.2,9.9 | 67.2,9.4 67.2,9.1 64.6,9.1 64.2,8.7 | 64.2,8.7 61.3,8.7 59.3,6.7 55.6,6.7 55.6,8.8 | 55.8,9 57.1,10.3 | 57.1,10.3 57.2,10.4 | 57.2,10.4 67.2,10.4 | 66,10.3 67.1,10.3 67.2,10.4 | 67.2,10.4 68.3,10.4 68.6,10.1 68.6,9.1 67.5,9.1 67,8.6 60.7,8.6 | 60.2,8.9 59.9,8.9 59.3,8.3 59.3,8 59.1,7.8 59.4,7.8 60.4,8.8 | 61.4,8.9 61.3,8.9 59.3,6.9 59.3,7.1 | 55.7,8.7 56,9 | 56,9 56.2,9.2 | 56.2,9.2 56.6,9.6 | 56.6,9.6 56.8,9.8 | 56.9,9.9 57.3,10.3 65.9,10.3 66.1,10.1 65.8,10.1 | 57.2,10.1 65.8,10.1 | 65.8,10.1 66,9.9 56.9,9.9 | 56.9,9.9 56.8,9.8 | 56.8,9.8 66,9.8 66,9.6 56.6,9.6 | 56.6,9.6 56.6,9.5 56.5,9.4 66,9.4 65.9,9.3 56.2,9.3 56.2,9.2 | 56.2,9.2 64.6,9.2 64.2,8.8 61,8.8 | 60.4,8.8 56,8.8 56.2,9 60.9,9 | 61.1,9 64.3,9 | 59.3,7.1 59.3,7.2 60.7,8.6 | 60.7,8.6 61.1,9 | 61.1,9 60.9,9 | 60.9,9 59.4,7.5 59.4,7.7 60.6,8.9 60.3,8.9 59.2,7.8 59.2,8 60.1,8.9 59.8,8.9 59.1,8.2 | 60.4,8.8 61,8.8 | 61,8.8 61.1,8.9 | 61,8.8 59.3,7.1 | 64.2,8.7 67,8.7 67.5,9.2 67.5,10.1 67.4,10.2 | 67.4,10.2 68.3,10.2 | 67.4,10.2 65.9,10.2 64.5,8.8 66.8,8.8 67.4,9.4 67.4,9.9 67.3,10 66.1,10 66.1,9.5 65.3,9.5 64.7,8.9 67.1,8.9 67.4,9.2 67.4,10.1 66.5,10.1 66.3,9.9 66.3,9.5 | 66.3,9.5 66,9.2 66.3,9.2 | 66.3,9.2 67,9.2 67.2,9.4 | 67.2,9.4 67.2,9.8 | 67.2,9.8 67.2,9.9 | 67.2,9.9 66.5,9.9 66.4,9.8 66.4,9.3 66.3,9.2 | 66.3,9.2 66.3,9.3 66.5,9.5 67.1,9.5 67.1,9.4 66.3,9.4 66.3,9.5 | 66.3,9.5 66.6,9.8 67.2,9.8 | 56,9 55.8,9 | 55.8,9 55.6,8.8 | 55.6,8.8 55.5,8.7 54.3,8.7 | 54.3,8.7 54.1,8.5 | 54.1,8.5 53.8,8.2 53.8,6.7 56.3,6.7 56.4,6.8 54,6.8 53.9,6.9 53.9,7.7 | 53.9,7.7 53.9,8 54.3,8.4 | 54.3,8.4 54.5,8.6 | 54.6,8.6 55.1,8.6 | 55.1,8.6 56,8.6 | 54.5,8.6 54.4,8.6
  Bottom 0.2: 54.4,8.6 54,8.2 54,8 | 54,8 54,7.9 | 54,7.6 54,7.4 | 54,7.2 54,7 55.8,7 55.9,7.1 55.9,7.2 54,7.2 | 54,7.2 54,7.4 | 54,7.4 56.1,7.4 56.1,7.6 55.8,7.6 | 54,7.6 54,7.9 | 54,7.9 56.4,7.9 56.6,7.7 55.9,7.7 55.8,7.6 | 55.8,7.6 54,7.6 | 54,7.6 53.9,7.7 | 53.9,7.7 56.3,7.7 56.4,7.6 56.2,7.6 55.7,8.1 54.3,8.1 | 54.3,8.1 54.1,8.1 54,8 | 54,8 55.6,8 55.8,8.2 | 54.2,8.2 55.8,8.2 | 55.8,8.2 56,8.4 54.8,8.4 | 54.6,8.4 54.3,8.4 | 54.3,8.3 54.3,8.7 | 54.3,8.1 54.3,8.3 | 54.3,8.3 54.1,8.5 | 54.3,8.7 56,10.4 56.3,10.4 | 57.2,10.4 56.3,10.4 | 56.3,10.4 56.2,10.3 56.1,10.3 54.4,8.6 | 54.5,8.6 54.6,8.6 | 54.6,8.6 56.3,10.3 56.5,10.3 | 57.1,10.3 56.8,10.3 | 56.7,10.3 56.5,10.3 | 56.5,10.3 54.6,8.4 | 54.6,8.4 54.8,8.4 | 54.8,8.4 56.7,10.3 | 56.7,10.3 56.8,10.3 | 56.8,10.3 56.9,10.2 56.7,10.2 55.1,8.6
N$117
  Bottom 0.2: 21.3,18.3 21.3,18.2 21.7,17.8
N$118
  Bottom 0.2: 39.2,5.4 39.2,5.6 37.4,5.6 | 37.4,5.6 37.3,5.7 | 37.4,5.6 37.5,5.5 38.9,5.5 39,5.4 38,5.4 37.9,5.3 38.9,5.3
N$119
  Bottom 0.2: 22.7,0.3 22.6,0.3 20.5,0.4
N$120
  Bottom 0.2: 31,26.4 30.4,26.4 | 30.4,26.4 6.5,26.4 | 6.5,26.4 6,26.4 | 6,26.4 5.9,26.4 | 5.9,26.4 5.7,26.4 5.7,26.5 30.9,26.5 | 5.6,26.7 31.23,26.7 | 31.23,26.7 IC6.4 | 6.1,26.5 6.1,26.2 | 6.4,26.2 30.7,26.2 | 30.7,26.2 31,26.2 31,25.8 | 31,25.8 31,22.2 | 31,22.2 31.5,22.2 | 31.5,22.2 31.5,26.7 31.4,26.7 | 31.4,26.7 31.3,26.6 31.3,26.7 | 31.3,26.7 31.23,26.7 | 31.3,26.7 31.4,26.7 | 31.4,26.7 31.4,26.6 31.3,26.5 31.3,22.4 31.5,22.2 | 31.5,22.2 31.5,22.1 | 31.5,22.1 31.5,22 | 31.5,22 31.4,22 | 31.4,22 30.9,22 | 30.9,22 30.9,26.5 | 30.9,26.5 30.9,26.6 31,26.6 31.1,26.5 31.1,25.8 | 31.1,25.8 31.1,22.4 31.2,22.3 | 6,26.4 5.9,26.3 5.9,25.8 6.5,26.4 | 5.9,26.6 5.7,26.6 5.6,26.7 | 5.6,26.7 5.5,26.7 | 30.9,22 30.9,21.7 | 30.9,21.7 31.5,21.7 | 31.5,21.7 31.5,22 | 31.5,22.1 31.3,22.1 31.1,21.9 | 31,22.2 31,21.9 31.1,21.8 31.4,21.8 | 31.4,22 31.4,21.8 | 31.4,21.8 31.5,21.7 | 31.5,21.7 31.5,21.6 30.9,21.6 30.9,21.7 | 31.1,25.8 30.7,26.2 | 30.4,26.4 31,25.8 | JP1.1 5.5,25.67 5.5,26.7 | 5.5,26.7 2.9,26.7 2.6,26.4 2.6,24.7 6.1,24.7 6.1,25.9 6.4,26.2 | 6.4,26.2 6.1,26.2 | 6.1,26.2 6,26.1 6,24.9 2.7,24.9 2.7,26.3 2.9,26.5 5.8,26.5 5.9,26.4 | 5.9,26.4 5.9,25.1 2.8,25.1 2.8,25.4 | 2.8,26.1 2.8,26.2 3,26.4 5.6,26.4 5.8,26.2 5.8,25.3 5.7,25.2 3,25.2 2.9,25.3 | 2.8,26 2.8,26.1 | 2.8,26.1 2.9,26.2 5.5,26.2 5.6,26.3 5.6,26 5.7,25.9 5.7,25.3 2.9,25.3 | 2.9,25.3 2.8,25.4 | 2.8,25.4 2.8,25.5 | 2.8,25.9 2.8,26 | 2.8,26 2.9,26.1 5.4,26.1 5.5,26 | 5.6,25.8 5.6,25.6 5.5,25.5 2.8,25.5 | 2.8,25.5 2.8,25.9 | 2.8,25.9 2.9,26 5.5,26 | 5.5,26 5.6,25.9 5.6,25.8 | 5.6,25.8 2.9,25.8 2.9,25.6 4.9,25.6 5,25.7 5.3,25.7 5.6,25.4
N$121
  Bottom 0.2: 2.7,21 2.9,21 2.9,14.6 2.4,15.1 2.4,21 2.7,21 | 2.7,21 2.8,20.9 2.8,14.8 | 2.8,14.8 2.9,14.7 | 2.8,14.8 2.5,15.1 2.5,20.8 2.6,20.9 2.6,15.2 2.7,15.1
N$123
  Bottom 0.2: 13.8,14.7 13.8,15.4 3.5,15.4 3.5,14.7 | 13.8,14.7 3.5,14.7 | 3.5,14.7 3.5,14.6 13.8,14.6 | 13.8,14.6 13.7,15 13.8,15.2 3.7,15.3 3.6,15.2 3.6,15.1 13.8,15.1 13.6,14.9 3.7,14.9 3.6,14.8 3.6,14.9 3.7,15 | 13.8,14.7 13.8,14.6
N$124  (via drill 0.6)
  Top 0.2: v44.3,11.4 2.1,11.4 v2.1,6.8
  Bottom 0.05: v2.1,6.8 JP7.1
  Bottom 0.2: 43.7,10.9 43.7,10.8 | 43.7,10.8 43.9,10.6 45.2,10.6 45.2,10.7 | IC6.10 37.9,13.31 | 37.9,13.31 37.9,11.9 | 37.9,11.9 37.9,11.4 v44.3,11.4 | 37.9,14.3 37.9,14.6 37.7,14.8 37.3,14.8 37.3,11.4 37.4,11.3 | 37.6,11.1 43.4,11.1 | 43.6,11.1 44.9,11.1 44.9,11.8 | 44.9,11.8 42.1,11.8 42,11.7 38.1,11.7 37.9,11.9 | 37.9,13.31 37.9,14.3 | 37.9,14.3 37.7,14.5 | 37.7,14.5 37.5,14.7 37.5,11.4 37.7,11.2 44.7,11.2 | 44.7,11.2 44.7,11.5 | 44.7,11.5 37.8,11.5 37.7,11.4 44.5,11.4 44.7,11.2 | 44.7,11.5 44.7,11.6 37.7,11.6 | 37.7,11.6 37.7,14.5 | 37.7,14.7 37.7,14.5 | 37.7,11.6 37.6,11.5 | 44.9,11.8 45.2,11.8 45.2,10.7 | 45.2,10.7 43.8,10.7 43.4,11.1 | 43.4,11.1 43.6,11.1 | 43.6,11.1 43.8,10.9 45.1,10.9 45.1,11.2 | 45.1,11.6 45.1,11.2 | 45.1,11.2 45,11.1 45,11.7 | 37.4,11.6 37.4,11.3 | 37.4,11.3 37.6,11.1 | 37.6,11.1 37.7,11 43.5,11 43.7,10.8
N$125
  Bottom 0.2: 15.6,8.4 16.6,7.4 16.3,7.4 | 14.5,14 14.5,8.3 16.4,6.4 | 16.4,6.4 16.9,6.4 16.9,6.5 | 16.9,7.3 16.9,7.7 | 16.9,7.7 16.7,7.9 | 16.7,7.9 16.1,8.5 16.1,13.9 | 16.1,13.9 14.6,13.9 14.5,14 | 14.5,14 16.1,14 | 16.1,14 15.9,13.8 14.6,13.8 14.6,8.4 16.5,6.5 16.6,6.5 | 16.6,6.5 16.7,6.6 16.7,6.8 | 16.7,7 16.7,7.7 16.1,8.3 16.1,7.3 16.6,6.8 | 16.6,6.8 16.9,6.5 | 16.9,6.5 16.9,7.3 | 16.9,7.3 16.2,8 16.2,7.7 16.6,7.3 16.3,7.3 16.2,7.4 | 16.2,7.4 16.3,7.4 | 16.3,7.4 16.7,7 | 16.7,7 16.7,6.8 | 16.7,6.8 16.6,6.7 14.8,8.5 14.9,8.5 | 15.7,8.5 15.9,8.5 15.9,8.4 | 15.9,8.2 15.9,7.8 15.7,7.8 | 15.7,7.8 15.1,8.4 | 15.1,8.4 15.2,8.4 15.3,8.3 | 16.2,7.4 16.2,7.5 15.4,8.3 15.8,8.3 15.9,8.4 | 15.9,8.4 15.9,8.2 | 15.9,8.2 15.8,8.1 15.7,8.2 15.8,8.2 16,8.4 16,13.6 15.9,13.7 | 15.9,13.7 14.8,13.7 14.8,8.7 | 14.8,8.7 14.8,8.6 14.9,8.5 | 14.9,8.5 15.7,8.5 | 15.7,8.5 15.8,8.6 15.8,8.7 | 15.8,8.7 15.8,13.6 15.5,13.6 | 15.4,13.6 15.3,13.6 | 15.2,13.6 15,13.6 15,8.8 15.4,8.8 15.7,8.5 | 15.7,8.5 15.7,8.6 | 15.7,8.6 15.8,8.7 | 15.8,8.7 15.5,8.7 | 14.8,8.7 14.9,8.7 | 14.9,8.7 15.1,8.7 | 15.1,8.7 15.5,8.7 | 15.5,8.7 15.6,8.8 15.6,9.1 | 15.6,9.1 15.6,13.5 15.5,13.6 | 15.5,13.6 15.4,13.6 | 15.4,13.6 15.3,13.5 15.3,8.9 15.1,8.7 | 15.1,8.7 15.1,9.4 15.2,9.5 15.2,13.6 | 15.2,13.6 15.3,13.6 | 15.3,13.6 15.5,13.4 15.5,8.8 15.7,8.6 | 14.9,8.7 14.9,8.3 | 14.9,8.3 16.5,6.7 | 16.6,6.8 16.6,6.6 16.4,6.4 | 16.4,6.4 17.4,5.4 | 17.4,5.4 17.7,5.1 | 17.7,5.1 17.8,5.1 17.8,5.4 | 17.8,5.4 17,6.2 | 17,6.2 16.7,6.5 | 16.6,6.5 16.6,6.4 17.6,5.4 | 17.6,5.4 17.7,5.3 | 17.6,5.4 17.5,5.4 17.4,5.5 17.4,5.4 | 17.7,5.1 18,4.8 18,5.2 17.8,5.4 | 16.2,7.4 15.3,8.3 | 15.3,8.3 14.9,8.3 | 14.9,8.3 14.8,8.4 15.1,8.4 | 15.7,7.8 16.6,6.9 16.6,7.8 16.7,7.9
  Bottom 0.2: 16.9,7.7 17,7.6 17,6.2 | 15.6,9.1 17,7.7 | 16.1,14 16.1,13.9 | 16.1,13.9 15.9,13.7
N$126
  Bottom 0.15: 33.6,22.4 33.6,21.7 33.7,21.7 | 33.8,21.7 34,21.7 34,22.2 | 33.8,22.3 33.7,22.3 33.7,21.7 | 33.7,21.7 33.8,21.7 | 33.8,21.7 33.8,22.3 | 33.8,22.3 34,22.3 34,22.2 | 34,22.2 33.9,22.2 33.9,21.8
N$127
  Bottom 0.2: 1.5,9.6 1.5,8.6 | 1.5,8.6 1.5,8.5 2,8.5 2.1,8.6 2.1,8.7 | 2.1,9.5 2.1,9.6 2,9.6 | 1.4,9.6 2,9.6 | 2,9.6 2.1,9.5 | 2.1,9.5 2.1,8.7 | 2.1,8.7 2,8.6 1.9,8.6 1.7,8.8 | 1.6,8.9 1.6,8.7 1.8,8.7 2,8.9 2,9.2 | 2,9.2 2,9.4 1.9,9.5 1.7,9.5 1.6,9.4 1.6,8.9 | 1.6,8.9 1.7,8.8 | 1.7,8.8 1.7,9.3 1.8,9.4 1.8,9 | 1.8,8.9 1.8,9 | 1.8,9 2,9.2 | 2.3,9.8 2.3,8.4 1.3,8.4 | 1.3,8.4 1.3,9.8 2.2,9.8 | 1.5,8.6 1.3,8.4 | 1.3,8.4 0.7,8.4 0.7,9.8 1,9.8 | 1.2,9.8 1,9.8 | 1,9.8 0.9,9.7 | 0.9,9.7 0.9,8.5 1.1,8.5 1.1,9.6 1.2,9.7 0.9,9.7
N$129
  Bottom 0.2: 44.9,22 43.2,22 43.1,22.1 | 43.1,22.1 43,22.1 | 43.1,22.1 44.7,22.1 44.8,22.2
N$130
  Bottom 0.2: 19,5.2 20.1,5.2 | 20.1,5.2 20.1,5.1 20.5,4.7 20.5,4.5 20.6,4.4 20,4.4 19.9,4.5 | 19.9,4.5 19.9,4.6 19.4,5.1 19.9,5.1 20,5 | 20,5 20,4.9 20.4,4.5 20.2,4.5 19.7,5 19.7,4.7 19.9,4.5 | 20.1,5.2 20.6,4.7 20.4,4.7 20.1,5 20,5 | 20,5 19.9,4.9 19.9,4.7 20.1,4.5
N$131
  Bottom 0.2: 21.5,3.5 21.5,1.4 | 21.5,1.4 21.8,1.1 21.9,1 27.7,1 27.7,3.1 26.7,4.1 26.7,1.3 22.6,1.3 22.4,1.5 22.4,3 21.4,4 21.4,1.5 21.5,1.4
N$132
  Bottom 0.2: 21.5,3.7 22.3,2.9 22.3,1.2 21.9,1.2 21.6,1.5 21.6,3.4 22.2,2.8 22.2,1.5 22.1,1.4 22.1,1.3 22,1.3 21.8,1.5 21.8,3.1 21.9,3 21.9,1.5 22,1.4 22.4,1.4 22.5,1.3 22.5,1.2 22.4,1.1 27.6,1.1 27.6,3.1 26.9,3.8 26.9,1.3 26.8,1.2 27.4,1.2 27.5,1.3 27.5,3 27,3.5 27,1.4 27.1,1.3 27.2,1.3 27.3,1.4 | 27.3,1.4 27.3,3 27.1,3.2 27.1,2.7 27.1,2 | 27.1,2 27.1,1.5 27.2,1.4 27.3,1.4 | 27.3,1.4 27.4,1.3 27.3,1.3 27.3,2.4 27.2,2.5 | 27.1,2 26.3,1.2
N$133
  Bottom 0.2: 17.9,1.2 18,1.1 18,0.2 16.4,0.2 16.4,1.2 16.5,1.3 17.3,1.3 17.9,0.7 16.5,0.7 16.5,0.6 17.8,0.6 17.9,0.5 17.9,0.4 16.6,0.4 16.5,0.5 16.5,0.3
N$134
  Bottom 0.2: 14,1.5 14,0.2 15.6,0.2 15.6,1.1 14.4,1.1 14.1,0.8 14.1,0.3 15.4,0.3 15.5,0.4 15.5,0.6 15.4,0.7 15.4,0.8 14.5,0.8 | 14.5,0.8 14.3,0.8 14.2,0.7 14.2,0.5 15,0.5 | 15.4,0.5 15,0.5 | 15,0.5 14.8,0.7 14.7,0.7 14.6,0.6 | 14.6,0.6 15.3,0.6 | 14.6,0.6 14.4,0.6 | 14.5,0.8 14.3,0.6
N$135
  Bottom 0.2: 11.6,1.3 11.6,1 11.5,0.9 11.5,0.2 13.1,0.2 13.1,1 11.9,1 11.7,0.8 11.7,0.4 12.9,0.4 12.9,0.6 13,0.7 12,0.7 11.9,0.8 11.9,0.7 11.6,0.4 12.1,0.4 | 12.1,0.4 12.2,0.5 12.9,0.5 13,0.4 12.1,0.4 | 12.1,0.4 11.9,0.6 12,0.6 12.1,0.5
N$136
  Bottom 0.2: 10.5,1.3 10.5,1 10.6,0.9 10.6,0.2 9,0.2 9,0.8 10.4,0.8 10.5,0.7 10.5,0.4 9.1,0.4 9.1,0.6 10.4,0.6
N$137
  Bottom 0.2: 6.7,1.3 6.7,1.1 6.5,0.9 6.5,0.3 8,0.3 8.1,0.2 | 8.1,0.2 6.5,0.2 6.5,0.7 6.7,0.9 8.1,0.9 8.1,0.4 | 8.1,0.2 8.1,0.4 | 8.1,0.4 8,0.5 6.6,0.5 6.6,0.6 6.7,0.7 7.5,0.7 | 8,0.7 7.5,0.7 | 7.5,0.7 7.4,0.8
N$138
  Bottom 0.2: 3.9,1.3 3.9,0.3 | 3.9,0.3 3.9,0.2 5.5,0.2 5.5,0.8 4.1,0.8 4,0.7 4,0.5 5.3,0.5 5.4,0.6 4.2,0.6 4.1,0.7 4.1,0.5 3.9,0.3 | 3.9,0.3 5.2,0.3 5.4,0.5 5.4,0.3
N$139
  Bottom 0.2: JP2.1 34.5,9.6 | 34.5,9.6 34.4,9.5 34.1,9.5 33.9,9.7 | 33.9,9.7 34.2,9.7 34.3,9.6 34.5,9.6 | 34.5,9.6 34.7,9.4 | 34.7,9.4 35.2,9.4 35.2,11.2 | 35.2,11.2 35.3,11.3 | 35.3,11.3 35.1,11.3 34.9,11.1 34.9,9.5 35,9.5 35,11.1 34.9,11.2 34.9,10.7 34.7,10.5 34.7,10.1 34.8,10 34.8,11 35.2,11.4 35.2,12.4 35.1,12.5 35.1,13.25 IC6.12 | 35,13.2 35,13.4 34.8,13.6 34.8,15 35.3,15 35.3,12 | 35.2,12 34.8,12 | 34.8,12 34.8,14.7 35,14.9 35,12.2 34.9,12.1 35.1,12.1 35.2,12.2 35.2,14.8 35.1,14.9 | 34.8,12 34.8,11.7 33.6,10.5 33.6,9.5 | 33.6,9.5 33.6,9.4 | 33.6,9.4 34.5,9.4 | 34.5,10.7 34.5,11 | 34.5,11 34.5,11.2 35.3,12 | 35.3,12 35.2,12 | 35.2,12 35.1,11.9 | 34.1,10.9 35,11.8 | 35,11.8 35.1,11.9 | 35.1,11.9 35,11.9 35,11.8 | 35.3,12 35.3,11.8 | 35.3,11.5 35.3,11.3 | 35.2,11.2 34.7,10.7 34.7,9.4 | 34.7,9.4 34.5,9.4 | 34.5,9.4 34.5,10.7 | 34.5,10.7 35.3,11.5 | 35.3,11.5 35.3,11.8 | 35.3,11.8 34.5,11 | 35.3,11.3 35.3,9.2 | 35.3,9.2 33.7,9.2 33.6,9.3 | 33.6,9.3 33.6,9.4 | 33.9,9.7 33.8,9.7 33.6,9.5 | 33.6,9.3 33.6,8.3 35.3,8.3 35.3,9.2 | 35.3,9.2 35.2,9.3 33.9,9.3 33.7,9.1 33.7,8.9 | 33.7,8.7 33.7,8.5 35.2,8.5 35.2,8.7 33.7,8.7 | 33.7,8.7 33.7,8.9 | 33.7,8.9 35.2,8.9 35.2,9 33.8,9
N$141
  Bottom 0.2: 40,26.7 43.9,26.7 43.9,25.8 | 43.9,25.8 40.6,25.8 39.7,26.7 40,26.7 | 40,26.7 40.1,26.6 40.1,26.5 | 40.1,26.5 40.7,25.9 40.8,25.9 | 40.8,25.9 43.7,25.9 43.8,26 43.8,26.1 | 43.8,26.2 43.8,26.5 40.4,26.5 | 40.4,26.5 40.3,26.6 | 40.4,26.5 40.9,26 43.7,26 43.8,26.1 | 43.8,26.1 43.8,26.2 | 43.8,26.2 43.7,26.3 40.8,26.3 40.7,26.4 40.7,26.3 40.8,26.2 43.6,26.2 43.7,26.1 40.7,26.1 40.2,26.6 | 40.1,26.5 40,26.6 40,26.4 41.2,25.2 41.2,21.8 42.2,21.8 42.2,22.9 42.4,23.1 43.9,23.1 43.9,25.8 | 40.8,25.9 40.8,25.8 41.4,25.2 41.4,25.4 41.1,25.7
N$142
  Bottom 0.2: 52.8,8.5 52.8,8.1
N$143
  Bottom 0.2: 19.1,19.3 19.8,19.3 19.9,19.2
N$145
  Bottom 0.2: 57.9,26 57.7,26 57.4,26.3 57.4,26.6 59,26.6 59,26.4 58.9,26.3
N$146
  Bottom 0.2: 60.9,26.1 60.2,26.1 60,26.3 60,26.6 61.6,26.6 61.6,26.3 61.5,26.2
N$147
  Bottom 0.2: 62.9,26.1 62.8,26.1 62.6,26.3 62.6,26.6 64.2,26.6 64.2,26.3 64.1,26.2
N$148
  Bottom 0.2: 65.4,26.1 65.3,26.1 65,26.4 65,26.6 66.6,26.6 66.6,26.2
N$149
  Bottom 0.2: 70.1,6.3 73.2,6.3 | 73.2,6.3 73.2,0.2 | 73.2,0.2 70.4,0.2 70.4,6 70.1,6.3 | 70.1,6.3 70.1,0.2 71.4,0.2 71.9,0.7 | 73.2,6.3 73.5,6.3 73.5,0.2 73.2,0.2 | 73.2,0.2 73.3,0.3 73.3,6.1 73.4,6.2 73.4,0.3
N$150
  Bottom 0.2: 48.2,9.1 48.2,9.2 49.4,10.4 50,10.4 50.4,10.8 50.4,13.3 49.5,13.3
N$151
  Bottom 0.2: 32.6,17.6 32.6,19.2 32.5,19.3 33.1,18.8 33.3,18.9 32.4,19.1 32.5,19 32.5,18.5 | 32.5,18.3 32.5,18.1 | 32.5,17.9 32.5,17.7 33.9,18.2 33.5,17.9 32.5,17.9 | 32.5,17.9 32.5,18.1 | 32.5,18.1 33.4,17.8 33.1,17.6 32.5,18.3 | 32.5,18.3 32.5,18.5 | 32.5,18.5 32,19 32.1,19 32.4,18.7 32.4,18.8 32.2,19 32.4,19.2
N$152
  Bottom 0.2: 43.1,15.9 44.4,15.9 | 44.4,15.9 48.4,15.9 48.4,16 48.3,16.1 44.6,16.1 44.4,15.9
N$154
  Bottom 0.2: 34,11.9 34,11.8 33.7,11.5 33.6,11.5 | 31.7,11.1 32.2,11.1 32.3,11 32.3,10.2 | 32.3,10.2 32.3,10 32.1,9.8 | 32.1,10.7 32.1,10.9 32,11 32,10 31.9,9.9 | 31.9,9.9 31.9,10.7 32.2,11 | 32.1,9.8 32.1,10.7 | 32.1,10.7 31.5,11.3 | 33.4,11.2 32.7,11.2 32.5,11 32.5,10.4 | 32.5,9.7 32.4,9.7 | 31.6,9.7 31.5,9.7 31.5,11.2 32,11.2 | 32.6,11.2 32.1,11.2 | 32.1,11.2 32,11.2 | 32,11.2 31.8,11 31.8,9.9 31.6,9.7 | 33.6,13.3 33.6,13.7 33.5,13.8 33.5,15 34.1,15 34.1,12 | 33.8,12 33.6,12 33.5,12.1 | 33.5,12.1 33.5,14.7 33.7,14.9 33.7,12.1 33.8,12.1 33.9,12.2 | 33.9,14.9 33.9,12.2 | 33.9,12.2 34,12.1 | 33.5,12.1 33.5,11.5 | 33.5,11.4 33.5,11.3 | 33.5,11.3 33.3,11.3 | 33.3,11.3 33.2,11.3 | 31.6,11.3 31.6,9.7 | 31.6,9.7 32.4,9.7 | 32.4,9.7 32.4,10.2 | 32.4,10.2 32.4,10.5 | 32.4,10.7 32.4,11.3 | 33.5,11.3 34.1,11.9 34.1,12 | 34.1,12 33.8,12 | 33.8,12 33.7,11.9 33.7,11.7 | 33.7,11.7 33.7,11.6 33.6,11.5 | 33.6,11.5 33.5,11.4 | 33.5,11.4 33.5,11.5 | 33.5,11.5 33.7,11.7 | 33.7,11.7 33.9,11.9 | 33.7,11.7 33.6,11.7 33.4,11.5 | 32.4,11.3 32,11.3 | 32,11.3 31.6,11.3 | 31.6,11.3 31.5,11.3 | 31.5,11.3 31.5,9.4 | 31.5,9.4 32.5,9.4 | 32.5,9.4 32.5,9.7 | 32.5,9.7 32.3,9.5 31.7,9.5 31.6,9.6 32,9.6 32.2,9.8 32.1,9.8 | 32.1,9.8 32,9.9 31.9,9.9 | 33.6,11.5 33.4,11.5 | 33.4,11.5 33.2,11.3 | 33.2,11.3 32.8,10.9 | 32.8,10.9 32.4,10.5 | 32.4,10.5 32.4,10.7 | 32.4,10.7 32.8,11.1 | 33.3,11.3 33.3,11.2 32.7,10.6 | 32.5,10.4 32.3,10.2 | 33.6,11.5 33.6,11.4 | 33.5,11.3 33.4,11.2 | 33.4,11.2 32.4,10.2 | 32.8,10.9 32.8,9.4 | 32.8,9.4 32.5,9.4 | 32.5,9.7 32.5,10.4 | 32.5,10.4 32.7,10.6 | 32.7,10.6 32.7,9.6 32.6,9.5 | 32.1,11.2 32,11.3 | 31.5,11.3 31.3,11.3 | 31.3,11.3 31.2,11.2 | 31.2,11.2 31.2,9.4 31.3,9.4 | 31.3,9.4 31.5,9.4
  Bottom 0.2: 31.5,9.4 31.4,9.5 31.4,10 | 31.4,10 31.4,11.2 31.3,11.3 | 31.3,11.3 31.2,11.3 31.2,11.2 | 32.4,11.3 33.2,11.3 | 32.8,9.4 32.8,9.2 | 31.3,9.2 31.2,9.2 | 31.2,9.2 31.2,9.8 31.4,10 | 31.3,9.4 31.3,9.3 31.2,9.2 | 31.2,9.2 31.2,9.1 | 31.2,8.6 31.2,8.3 32.8,8.3 32.8,9.2 | 32.8,9.2 31.3,9.2 | 31.3,9.2 31.2,9.1 | 31.2,9.1 31.2,8.6 | 31.2,8.6 31.4,8.4 32.6,8.4 32.7,8.5 32.7,8.7 | 32.7,8.9 32.7,9 31.4,9 31.4,8.9 31.3,8.8 32.6,8.8 32.7,8.9 | 32.7,8.9 32.7,8.7 | 32.7,8.7 31.3,8.7 31.3,8.6 32.6,8.6
N$155
  Bottom 0.2: 62.8,7.8 67.1,7.8 67.4,8.1 68.6,8.1 68.6,7.1 67.9,6.4 67.9,1.8 67.8,1.7 | 67.8,1.7 67.7,1.6 62.9,1.6 62.6,1.9 62.6,7.8 67.4,7.8 | 67.4,7.8 67.5,7.9 | 67.5,7.9 67.5,7.8 67.7,7.6 | 68,7.3 68.3,7 68.2,7 67.7,6.5 67.7,7 67.2,7.5 | 67.2,7.5 67,7.7 67,6.4 67.7,6.4 67.8,6.5 | 67.8,6.5 67.9,6.6 | 67.9,6.6 67.9,7.7 67.8,7.8 67.4,7.8 | 67.4,7.8 67.3,7.7 67.5,7.7 67.6,7.6 67.7,7.6 | 67.7,7.6 68,7.3 | 68,7.3 67.8,7.3 | 67.8,7.3 67.6,7.3 67.2,7.7 | 62.9,1.7 67.8,1.7 | 67.2,7.5 67.2,7.7 | 67.2,7.7 67.5,8 67.5,7.9 | 67.5,7.9 68.3,7.1 68.2,7.1 68,6.9 68,6.7 67.9,6.6 | 67.8,6.5 67.9,6.5 68.3,6.9 68.2,6.9 67.8,7.3
N$156
  Bottom 0.2: 59.5,5.5 59.5,5.7 61.6,7.8 61.8,7.8 61.8,1.5 58.7,1.5 58.7,5.7 61.7,5.7 61.7,7.7 59.8,5.8 61.5,5.8 61.5,7.2 | 61.5,7.2 61.5,7.3 61.6,7.4 61.5,7.4 60,5.9 61.3,5.9 61.4,6 61.4,7.1 | 61.4,7.1 61.5,7.2 | 61.4,7.1 60.3,6 61.2,6 61.3,6.1 61.3,6.7 61.2,6.8 61.2,6.7 | 61.2,6.7 60.6,6.1 61.1,6.1 61.2,6.2 61.2,6.3 | 61.2,6.3 61.2,6.5 | 61.2,6.7 61.2,6.5 | 61.2,6.5 60.9,6.2 61.1,6.2 61.2,6.3
N$157
  Bottom 0.2: 34.4,9.9 34.4,9.5 33.8,9.5 33.8,10.5 34.4,11.1 34.4,10.7 | 34.4,10.7 34.4,9.9 | 34.4,9.9 34.2,9.7 34.2,10.7 | 34.2,10.7 34.3,10.8 | 34.2,10.7 34,10.5 34,9.8 | 35.1,11.5 35.1,11.4 34.4,10.7
N$158
  Bottom 0.2: 54.6,5.4 54.6,5.5 54.4,5.7 | 54.4,5.7 54,5.7 | 54.4,5.7 57.4,5.7 57.4,1.5 53.9,1.5 53.9,5.7
N$159
  Bottom 0.2: 73.3,25 73.3,21 | 73.3,21 73.3,19.4 73.3,19 73.3,15.6 73,15.9 73,21.3 73.3,21
N$161
  Bottom 0.2: 14.3,18.7 14.4,18.5
N$162
  Bottom 0.2: 13.8,18.8 14.2,18.3
N$163
  Bottom 0.2: IC6.13 33.8,13.31 33.8,11.8 33.6,11.8 32.6,10.8 32.2,10.8 JP3.1
N$164
  Bottom 0.2: 49.1,16 49.4,16
N$165
  Bottom 0.2: 48.4,16.6 47.8,16
N$166
  Bottom 0.2: 48.6,16.9 47.7,16
N$167
  Bottom 0.2: 42.4,23.4 42,23 42.2,23 42.5,23.3
N$168
  Bottom 0.2: 16.9,14.2 16.9,13.6
N$169
  Bottom 0.2: 16.7,16.6 16.2,16.1 16.2,15.8 16.3,15.7 19.2,15.7 19.6,16.1 29.2,16.1 29.6,15.7 | 29.7,13.1 29.7,12.1 | 29.7,12.1 30.3,12.1 30.3,12.3 | Q1.1 20.6,16.4 | 20.8,16.4 29.2,16.4 | 29.2,16.4 29.3,16.4 | 29.3,16.4 30,15.7 | 30,15.7 30,13.35 IC6.16 | 30.3,15.4 30,15.7 | 30,15.7 29.9,15.7 29.8,15.6 29.8,12.2 29.7,12.1 | 29.7,12.1 29.6,12.1 29.6,15.7 | 29.6,15.7 29.6,15.9 | 29.6,15.9 29.2,16.3 29.2,16.4 | 29.3,16.4 29.7,16.4 30.3,15.8 | 30.3,15.8 30.3,15.4 | 30.3,15.4 30.3,12.3 | 30.3,12.3 30.2,12.2 30.1,12.2 | 30.1,12.2 30,12.3 30,15.8 29.6,16.2 29.7,16.2 30.1,15.8 | 30.1,15.8 30.2,15.7 29.8,15.7 29.7,15.8 29.7,12.4 29.9,12.2 30.1,12.2 | 30.1,12.2 30.2,12.3 30.2,15.3 30.1,15.4 | 29.6,15.9 29.6,16 29.4,16.2 19.5,16.2 | 19.5,16.2 16.9,16.2 | 16.9,16.2 16.7,16.4 16.3,16 16.3,15.9 16.4,15.8 19.1,15.8 19.5,16.2 | 16.9,16.2 16.7,16.2 16.6,16.1 | 16.6,16.1 19.2,16.1 19,15.9 16.4,15.9 16.6,16.1 | 16.8,16.5 16.7,16.6 | 16.7,16.6 16.8,16.7 20.5,16.7 | 20.5,16.7 20.7,16.5 | 20.7,16.5 20.8,16.4 | 20.8,16.4 20.6,16.4 | 20.6,16.4 20.4,16.6 19.1,16.6 19,16.5 | 20.5,16.7 30.3,16.7 30.3,15.8 | 30.3,15.4 30.2,15.4 30.2,16.6 20.7,16.6 20.7,16.5 | 20.7,16.5 30.1,16.5 30.1,15.8 | 30.1,15.8 29.9,15.8 29.9,16.4
N$170  (1 unrouted)
  Bottom 0.2: 14.4,19.8 14.4,20.5 15,21.1 19.2,21.1 | 46.1,7.8 46.1,11.3 | 46.1,11.5 46.1,11.8 | 46.1,11.8 46.1,12.4 48.8,12.4 | 14.3,18.4 14.3,17.5 | 14.3,18.8 14.4,18.8 14.4,18.6 | 14.3,22 14.3,18.8 | 41.8,12.7 48.3,12.7 | 48.3,12.7 49.1,12.7 | 49.1,12.7 49.2,12.7 | 49.2,12.7 49.4,12.7 | 49.4,12.7 50,12.7 50,11.3 50.1,11.2 49.5,10.6 | 49.4,10.5 45.5,6.6 45.5,6.8 45.6,6.9 | 45.7,7 49.9,11.2 49.8,11.2 | 49.8,11.2 49.6,11.2 | 49.6,11.2 45.3,6.9 46.1,6.9 49.8,10.6 49.5,10.6 | 49.5,10.6 49.4,10.5 | 49.4,10.5 49.4,10.8 49.6,11 49.5,11 49.4,10.9 | 49.4,10.9 45.9,7.4 | 17.5,14.2 17.4,14.1 | 17.4,14.1 17.4,14.2 17.9,14.7 18.3,14.7 | 18.3,14.7 19.7,14.7 | 14.5,17.4 14.5,17.5 | 14.5,18.5 14.4,18.6 | 45.5,15.9 45,16.1 43,16.1 43,15.8 43.4,15.4 47.9,15.4 | 43.1,7.5 43.2,7.4 | 43.5,7.1 43.6,7 | 43.8,6.8 44.2,6.4 | 44.2,6.4 44.3,6.3 44.3,6.6 | 44.6,6.9 44.6,6.6 44.4,6.8 44.2,6.8 43.9,7.1 | 44.6,7.4 44.6,7.6 | 44.8,6.6 44.2,6.6 43.3,7.5 | 43.8,7.2 43.7,7.3 | 43.7,7.3 43.4,7.6 46.5,7.6 | 69.1,1 69,1 68.5,0.5 | 20.5,3.9 20.5,4.1 20.7,4.3 20.7,4.8 20.1,5.4 18.8,5.4 18.7,5.5 | 68.2,13.3 68.2,17.3 68,17.3 | 17,13.8 17.1,13.9 17.1,14 | 50.1,10.6 45.6,6.1 45.6,2.3 | 50.1,10.6 49.9,11.3 50,12 | 50,12 49.7,12.7 | 50.2,12.9 49.7,12.7 | 49.7,12.7 50.3,13.1 | 50.3,13.1 41.3,13.1 41.3,12.9 50.2,12.9 | 50.2,12.9 49.8,12.7 50.1,11.3 46.8,7.6 | 46.8,7.6 45.9,6.7 | 45.9,6.7 45.3,6.1 | 50.3,13.1 50,12 | 45.5,2.5 45.5,2.3 | 45.5,2.3 45.6,2.3 | 45.6,2.3 46,2.3 | 46,2.3 46,6.3 | 46,2.3 46.2,2.3 46.2,6.4 46.1,6.5 | 32.2,14.5 32.2,12.1 32.8,12.1 32.8,15.3 33.2,15.7 | IC2.16 13.2,17.97 | 13.2,17.97 13.2,16 | 17.7,14.7 17.7,14.8 19.7,14.8 19.8,14.7 | 17.7,14.7 17.7,14.1 | 17.7,14.1 18.5,14.1 | 18.5,14.1 19.9,14.1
